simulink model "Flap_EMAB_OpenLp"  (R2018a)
settings: Solver=ode45  StartTime=0.0  StopTime=1  RelTol=1e-3  EnableMultiTasking=on
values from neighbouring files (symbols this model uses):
  Be = 25    [init.m]
  Ja = 2.0e-4    (= 0.0002)    [init.m]
  Je = 2.2    [init.m]
  Jm = 5.0e-5    (= 5e-05)    [init.m]
  Kdmp = 0.001    [init.m]
  Keff = 0.85    [init.m]
  Kgs = 400.0    (= 400)    [init.m]
  Ki = 5.0    (= 5)    [init.m]
  Kl = 12/Kli    (= 1800000)    [init.m]
  Kmfr = 0.03    [init.m]
  Kp = 140    [init.m]
  Krfb = 0.0005    [init.m]
  Kt = 12/Kti    (= 1674418.60465)    [init.m]
  Kv = 260    [init.m]
  Ngear = 10.2    [init.m]
  Nscrew = 0.0026    [init.m]
  R = 0.287    [init.m]    (also in lqr_des.m = diag(R))
  Wmb = 1500    [init.m]

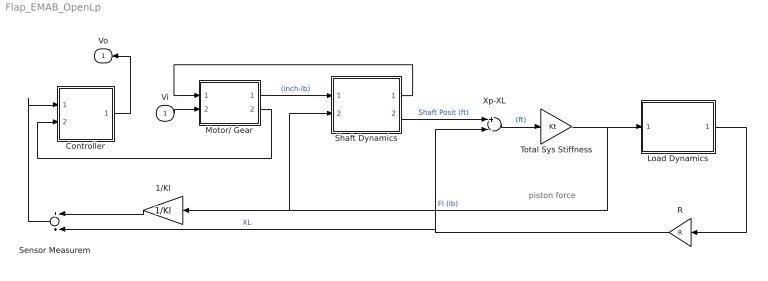
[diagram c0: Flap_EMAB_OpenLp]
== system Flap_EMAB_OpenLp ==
  note: piston force
  Vi : Inport
  1/Kl : Gain  Gain=1/Kl
  Controller : Subsystem
  Load Dynamics : Subsystem
  Motor/ Gear : Subsystem
  R : Gain  Gain=R
  Sensor Measurem : Sum
  Shaft Dynamics : Subsystem
  Total Sys Stiffness : Gain  Gain=Kt
  Xp-XL : Sum  Inputs=+-
  Vo : Outport
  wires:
  Shaft Dynamics/2(Xp) -> Xp-XL/1  "Shaft Posit (ft)"
  Xp-XL/1 -> Total Sys Stiffness/1  "(ft)"
  Total Sys Stiffness/1 -> Load Dynamics/1(FL), Shaft Dynamics/2(FL), 1/Kl/1  "Fl (lb)"
  1/Kl/1 -> Sensor Measurem/1
  Motor/ Gear/1(Tm) -> Shaft Dynamics/1(Tq-mot)  "(inch-lb)"
  Load Dynamics/1(Delta (rad)) -> R/1
  Shaft Dynamics/1(Xp-dot) -> Motor/ Gear/1(Xp-dot)
  R/1 -> Sensor Measurem/2, Xp-XL/2  "XL"
  Motor/ Gear/2(mr) -> Controller/2(rotor)
  Vi/1 -> Motor/ Gear/2(Vin)
  Sensor Measurem/1 -> Controller/1(Xp-fb)
  Controller/1(V) -> Vo/1

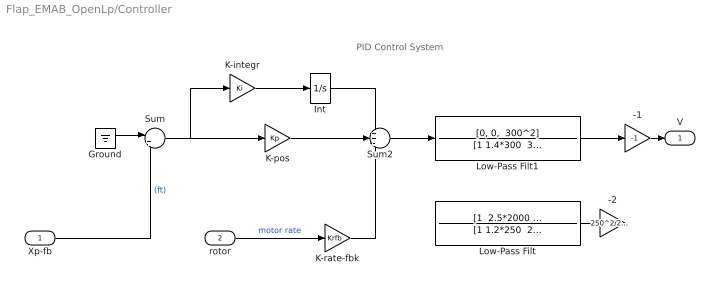
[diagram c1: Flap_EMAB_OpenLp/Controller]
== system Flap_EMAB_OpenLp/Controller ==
  note: PID Control System
  Xp-fb : Inport
  rotor : Inport  Port=2
  -1 : Gain  Gain=-1
  -2 : Gain  Gain=250^2/2000^2
  Ground : Ground
  Int : Integrator  UpperSaturationLimit=1  LowerSaturationLimit=-1
  K-integr : Gain  Gain=Ki
  K-pos : Gain  Gain=Kp
  K-rate-fbk : Gain  Gain=Krfb
  Low-Pass Filt : TransferFcn  Numerator="[1  2.5*2000  2000^2]"  Denominator="[1 1.2*250  250^2]"
  Low-Pass Filt1 : TransferFcn  Numerator="[0, 0,  300^2]"  Denominator="[1 1.4*300  300^2]"
  Sum : Sum  Inputs=|+-
  Sum2 : Sum  Inputs=++-
  V : Outport
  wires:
  Xp-fb/1 -> Sum/2  "(ft)"
  Sum/1 -> K-pos/1, K-integr/1
  rotor/1 -> K-rate-fbk/1  "motor rate"
  K-pos/1 -> Sum2/2
  K-integr/1 -> Int/1
  Int/1 -> Sum2/1
  K-rate-fbk/1 -> Sum2/3
  -1/1 -> V/1
  Ground/1 -> Sum/1
  Sum2/1 -> Low-Pass Filt1/1
  Low-Pass Filt/1 -> -2/1
  Low-Pass Filt1/1 -> -1/1

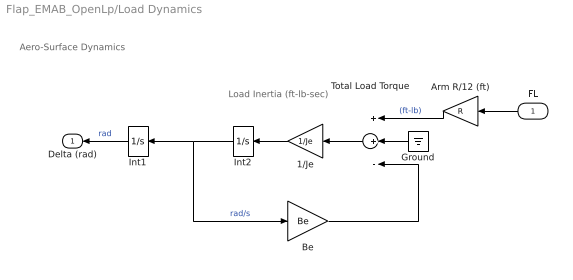
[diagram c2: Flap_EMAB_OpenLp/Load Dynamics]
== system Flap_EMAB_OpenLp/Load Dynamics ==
  note: Load Inertia (ft-lb-sec)
  note: Aero-Surface Dynamics
  FL : Inport
  1/Je : Gain  Gain=1/Je
  Arm R/12 (ft) : Gain  Gain=R
  Be : Gain  Gain=Be
  Ground : Ground
  Int1 : Integrator
  Int2 : Integrator
  Total Load Torque : Sum  Inputs=++-
  Delta (rad) : Outport
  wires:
  Ground/1 -> Total Load Torque/2
  Arm R/12 (ft)/1 -> Total Load Torque/1  "(ft-lb)"
  FL/1 -> Arm R/12 (ft)/1
  1/Je/1 -> Int2/1
  Int2/1 -> Int1/1, Be/1  "rad/s"
  Int1/1 -> Delta (rad)/1  "rad"
  Total Load Torque/1 -> 1/Je/1
  Be/1 -> Total Load Torque/3

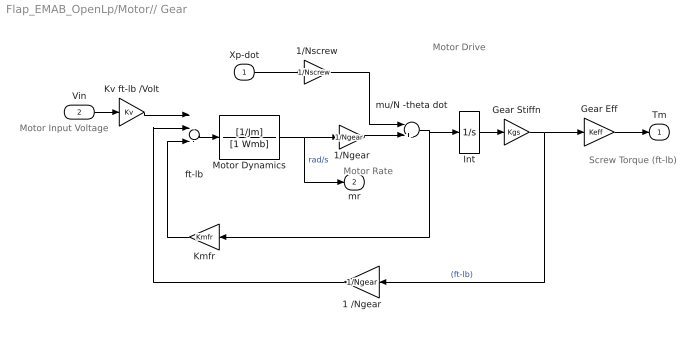
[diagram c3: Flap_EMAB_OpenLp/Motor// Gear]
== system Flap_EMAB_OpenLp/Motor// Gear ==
  note: Screw Torque (ft-lb)
  note: Motor Rate
  note: Motor Input Voltage
  note: Motor Drive
  Xp-dot : Inport
  Vin : Inport  Port=2
  1 /Ngear : Gain  Gain=1/Ngear
  1/Ngear : Gain  Gain=1/Ngear
  1/Nscrew : Gain  Gain=1/Nscrew
  Gear Eff : Gain  Gain=Keff
  Gear Stiffn : Gain  Gain=Kgs
  Int : Integrator  UpperSaturationLimit=0.4  LowerSaturationLimit=-0.4
  Kmfr : Gain  Gain=Kmfr
  Kv ft-lb /Volt : Gain  Gain=Kv
  Motor Dynamics : TransferFcn  Numerator=[1/Jm]  Denominator=[1 Wmb]
  ft-lb : Sum  Inputs=+---
  mu/N -theta dot : Sum  Inputs=-+
  Tm : Outport
  mr : Outport  Port=2
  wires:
  Int/1 -> Gear Stiffn/1
  Kmfr/1 -> ft-lb/3
  1/Nscrew/1 -> mu/N -theta dot/1
  Kv ft-lb /Volt/1 -> ft-lb/1
  Gear Eff/1 -> Tm/1
  Vin/1 -> Kv ft-lb /Volt/1
  Xp-dot/1 -> 1/Nscrew/1
  Gear Stiffn/1 -> Gear Eff/1, 1 /Ngear/1  "(ft-lb)"
  1/Ngear/1 -> mu/N -theta dot/2
  Motor Dynamics/1 -> mr/1, 1/Ngear/1  "rad/s"
  1 /Ngear/1 -> ft-lb/2
  ft-lb/1 -> Motor Dynamics/1
  mu/N -theta dot/1 -> Kmfr/1, Int/1

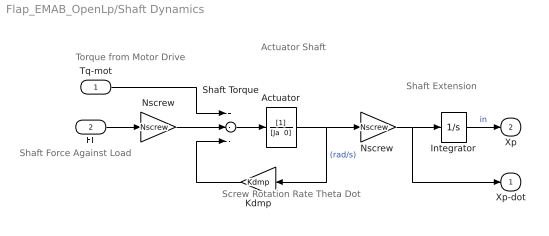
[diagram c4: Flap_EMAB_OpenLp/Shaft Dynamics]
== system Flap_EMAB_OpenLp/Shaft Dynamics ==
  note: Shaft Extension
  note: Screw Rotation Rate Theta Dot
  note: Shaft Force Against Load
  note: Torque from Motor Drive
  note: Actuator Shaft
  Tq-mot : Inport
  FL : Inport  Port=2
  Actuator : TransferFcn  Denominator="[Ja  0]"
  Integrator : Integrator
  Kdmp : Gain  Gain=Kdmp
  Nscrew : Gain  Gain=Nscrew
  "Nscrew " : Gain  Gain=Nscrew
  Shaft Torque : Sum  Inputs=+--
  Xp-dot : Outport
  Xp : Outport  Port=2
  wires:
  Kdmp/1 -> Shaft Torque/3
  "Nscrew "/1 -> Xp-dot/1, Integrator/1
  Nscrew/1 -> Shaft Torque/2
  FL/1 -> Nscrew/1
  Integrator/1 -> Xp/1  "in"
  Tq-mot/1 -> Shaft Torque/1
  Shaft Torque/1 -> Actuator/1
  Actuator/1 -> Kdmp/1, "Nscrew "/1  "(rad/s)"
